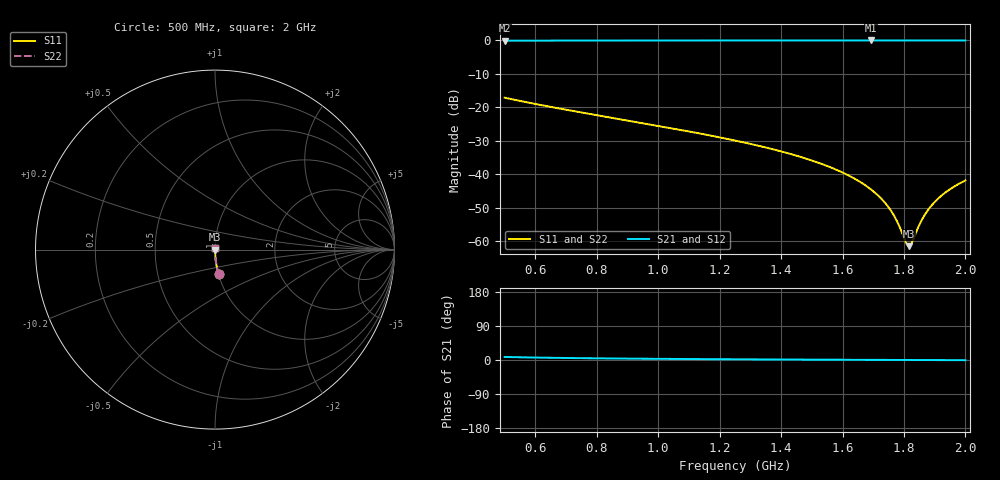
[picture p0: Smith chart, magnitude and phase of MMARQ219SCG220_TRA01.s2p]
! MMARQ219SCG220_TRA01  S-PARAMETER MODEL  ( General Type )
! Model Generated by TAIYO YUDEN Corporation (http://www.ty-top.com)
! Version 1.0
! TAIYO YUDEN Control No. 150609
! Copyright(c) 2015 TAIYO YUDEN CO.,LTD. All Rights Reserved.
! Product Description (link to TY-COMPAS)
! https://ds.yuden.co.jp/TYCOMPAS/or/detail?pn=MMARQ219SCG220JTRA01&u=M
! Products Name : Multilayer Ceramic Capacitors
! Characteristics :
!  Capacitance : 22 pF , Rated Voltage : 250V , TCC : CG / C0G
!  Case Size : 2.0 x 1.25 / 0.079 x 0.049 [mm/inch] , Thickness : 0.85 / 0.033 [mm/inch]
!  (Conditions: Temperature = 25 degC , DC Bias Current/Voltage = 0A / 0V)
! External Node Assignments :
!  1  o---| |---o  2
! GND o---------o GND
! Frequency Range : 500MHz  -  2GHz  [ 401 STEP ]
# MHz S RI R 50
! Freq[MHz].  S11 Real  S11 Imag  S21 Real  S21 Imag  S12 Real  S12 Imag  S22 Real  S22 Imag
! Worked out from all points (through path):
!   401 points, 500 MHz to 2 GHz, reference 50 ohm
!   highest |S21| = -0.01 dB at 1.692 GHz (marker M1); lowest = -0.1 dB at 500 MHz (marker M2)
!   group delay of S21, straight-line fit = 13.7 ps
!   lowest |S11| = -61.5 dB at 1.816 GHz (marker M3), VSWR 1.00, Z = 50.1 - j0.00045 ohm
!   |S11| at or under -10 dB: start of sweep to end of sweep
!   |S22| runs from -61.5 to -17.1 dB; largest |S21 - S12| = 0
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500  0.0198 -0.1381  0.9802 0.1381  0.9802 0.1381  0.0198 -0.1381
751.25  0.00744 -0.0834  0.9926 0.0834  0.9926 0.0834  0.00744 -0.0834
1002.5  0.00332 -0.0526  0.9967 0.0526  0.9967 0.0526  0.00332 -0.0526
1250  0.00168 -0.0319  0.9983 0.0319  0.9983 0.0319  0.00168 -0.0319
1388.75  0.00122 -0.0227  0.9988 0.0227  0.9988 0.0227  0.00122 -0.0227
1501.25  0.00101 -0.016  0.999 0.016  0.999 0.016  0.00101 -0.016
1610  0.000887 -0.0101  0.9991 0.0101  0.9991 0.0101  0.000887 -0.0101
1655  0.000859 -0.00777  0.9991 0.00777  0.9991 0.00777  0.000859 -0.00777
1692.5  0.000844 -0.00589  0.9992 0.00589  0.9992 0.00589  0.000844 -0.00589
1726.25  0.000837 -0.00424  0.9992 0.00424  0.9992 0.00424  0.000837 -0.00424
1752.5  0.000836 -0.00298  0.9992 0.00298  0.9992 0.00298  0.000836 -0.00298
1778.75  0.000837 -0.00174  0.9992 0.00174  0.9992 0.00174  0.000837 -0.00174
1805  0.000841 -0.000522  0.9992 0.000522  0.9992 0.000522  0.000841 -0.000522
1812.5  0.000843 -0.000177  0.9992 0.000177  0.9992 0.000177  0.000843 -0.000177
1816.25  0.000844 -4.49e-06  0.9992 4.49e-06  0.9992 4.49e-06  0.000844 -4.49e-06
1820  0.000845 0.000167  0.9992 -0.000167  0.9992 -0.000167  0.000845 0.000167
1827.5  0.000847 0.00051  0.9992 -0.00051  0.9992 -0.00051  0.000847 0.00051
1850  0.000855 0.00153  0.9991 -0.00153  0.9991 -0.00153  0.000855 0.00153
1865  0.000861 0.0022  0.9991 -0.0022  0.9991 -0.0022  0.000861 0.0022
1895  0.000876 0.00353  0.9991 -0.00353  0.9991 -0.00353  0.000876 0.00353
1943.75  0.000908 0.00565  0.9991 -0.00565  0.9991 -0.00565  0.000908 0.00565
2000  0.000953 0.00803  0.999 -0.00803  0.999 -0.00803  0.000953 0.00803
